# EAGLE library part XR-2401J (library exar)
MICROCONTROLLER
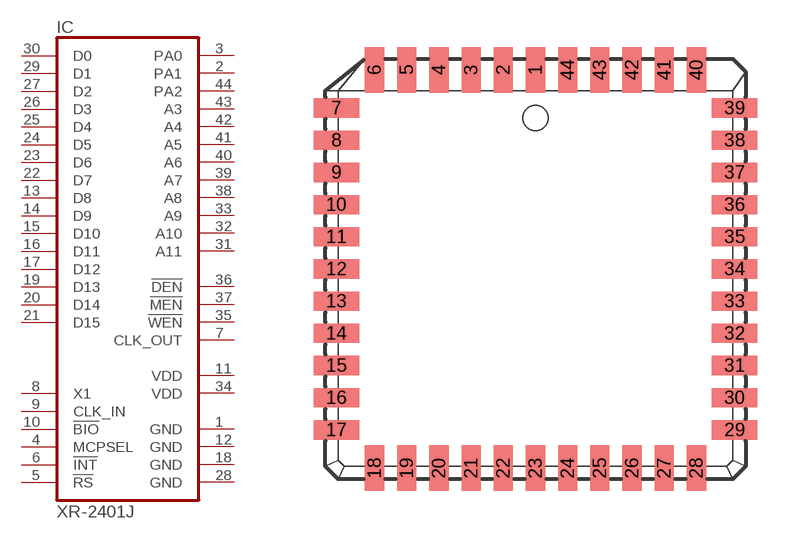
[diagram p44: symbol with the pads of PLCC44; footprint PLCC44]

Designator prefix IC

## XR-2401J (OC_FARNELL: unknown; OC_NEWARK: unknown)  [PLCC44]
1  GND  pwr
2  PA1  out
3  PA0  out
4  MCPSEL  in
5  !RS  in
6  !INT  in
7  CLK_OUT  out
8  X1  in
9  CLK_IN  in
10  !BIO  in
11  VDD  pwr
12  GND  pwr
13  D8
14  D9
15  D10
16  D11
17  D12
18  GND  pwr
19  D13
20  D14
21  D15
22  D7
23  D6
24  D5
25  D4
26  D3
27  D2
28  GND  pwr
29  D1
30  D0
31  A11  out
32  A10  out
33  A9  out
34  VDD  pwr
35  !WEN  out
36  !DEN  out
37  !MEN  out
38  A8  out
39  A7  out
40  A6  out
41  A5  out
42  A4  out
43  A3  out
44  PA2  out

## Footprint PLCC44 (pad centres in mm)
Plastic Leaded Chip Carrier
smd 0.76 x 1.8: 1 0,7.86; 2 -1.27,7.86; 3 -2.54,7.86; 4 -3.81,7.86; 5 -5.08,7.86; 6 -6.35,7.86; 18 -6.35,-7.86; 19 -5.08,-7.86; 20 -3.81,-7.86; 21 -2.54,-7.86; 22 -1.27,-7.86; 23 0,-7.86; 24 1.27,-7.86; 25 2.54,-7.86; 26 3.81,-7.86; 27 5.08,-7.86; 28 6.35,-7.86; 40 6.35,7.86; 41 5.08,7.86; 42 3.81,7.86; 43 2.54,7.86; 44 1.27,7.86
smd 1.8 x 0.76: 7 -7.86,6.35; 8 -7.86,5.08; 9 -7.86,3.81; 10 -7.86,2.54; 11 -7.86,1.27; 12 -7.86,0; 13 -7.86,-1.27; 14 -7.86,-2.54; 15 -7.86,-3.81; 16 -7.86,-5.08; 17 -7.86,-6.35; 29 7.86,-6.35; 30 7.86,-5.08; 31 7.86,-3.81; 32 7.86,-2.54; 33 7.86,-1.27; 34 7.86,0; 35 7.86,1.27; 36 7.86,2.54; 37 7.86,3.81; 38 7.86,5.08; 39 7.86,6.35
